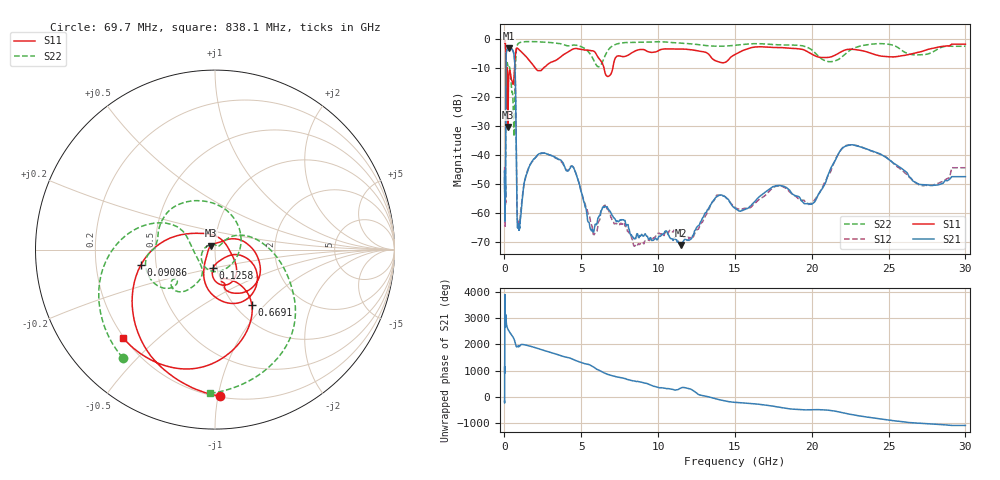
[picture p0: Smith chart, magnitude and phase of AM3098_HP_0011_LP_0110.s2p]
! Date/Time: Thu, Feb 28, 2019 8:34 AM
! Network Analyzer: Agilent Technologies E8364B Rev: A.07.50.67
! Sweep from 0.010 to 30.000 GHz, 1601 Points, Sweep Type: LOG
! Power Supply: 5.023 V, 0.002 A
# Hz S DB R 50
!freq MagS11 AngS11 MagS21 AngS21 MagS12 AngS12 MagS22 AngS22
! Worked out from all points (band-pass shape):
!   1601 points, 10 MHz to 30 GHz, reference 50 ohm
!   highest |S21| = -3.09 dB at 266.5 MHz (marker M1); lowest = -70.9 dB at 11.48 GHz (marker M2)
!   |S21| within 3 dB of the highest: 107.5 MHz to 640.8 MHz (533.3 MHz wide, 143 % of centre)
!   lowest |S11| = -30.2 dB at 227 MHz (marker M3), VSWR 1.06, Z = 47.8 + j2.13 ohm
!   |S11| at or under -10 dB: 176.1 MHz to 655.5 MHz (479.4 MHz wide, 115 % of centre); 2.028 GHz to 2.52 GHz (492.1 MHz wide, 21.6 % of centre); 6.485 GHz to 7.047 GHz (562.3 MHz wide, 8.31 % of centre)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
!   |S22| runs from -33.4 to -0.5 dB; largest |S21 - S12| = 0.011
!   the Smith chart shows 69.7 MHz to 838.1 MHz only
!   S11 on the Smith chart (normalised r, x): 69.7 MHz: 0.21, -1.01; 90.86 MHz: 0.41, -0.09; 125.8 MHz: 0.96, -0.20; 669.1 MHz: 1.19, -0.85; 838.1 MHz: 0.20, -0.39
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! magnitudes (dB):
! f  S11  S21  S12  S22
! 10 MHz  -0.3  -47.7  -46.0  -0.5
! 38.04 MHz  -0.5  -61.6  -61.4  -0.9
! 69.7 MHz  -1.8  -52.1  -54.6  -2.0
! 90.86 MHz  -7.5  -20.8  -20.7  -8.6
! 100.9 MHz  -23.6  -8.1  -8.2  -17.0
! 125.8 MHz  -19.9  -4.4  -4.4  -10.6
! 144.7 MHz  -14.1  -3.7  -3.7  -10.4
! 185.8 MHz  -11.2  -3.6  -3.5  -8.1
! 227 MHz  -30.2  -3.2  -3.2  -9.5
! 266.5 MHz  -14.6  -3.1  -3.1  -9.7
! 550.5 MHz  -15.5  -3.9  -3.9  -20.4
! 620.7 MHz  -13.1  -5.3  -5.2  -33.3
! 669.1 MHz  -8.7  -8.0  -8.0  -20.7
! 838.1 MHz  -3.0  -63.6  -61.5  -1.9
! 2.084 GHz  -10.4  -40.4  -40.4  -0.8
! 4.436 GHz  -3.3  -43.8  -43.8  -2.0
! 5.64 GHz  -3.8  -65.8  -63.8  -5.5
! 7.926 GHz  -5.7  -64.2  -64.8  -1.1
! 11.48 GHz  -3.3  -70.9  -66.9  -1.3
! 19.9 GHz  -4.8  -56.9  -56.6  -3.2
! 22.67 GHz  -3.4  -36.4  -36.4  -3.2
! 30 GHz  -1.6  -47.3  -44.3  -2.4
